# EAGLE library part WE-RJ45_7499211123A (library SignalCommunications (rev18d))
Order Code 7499211123A Design THT xBase-T 10/100 Base-T Ports 1x1 Application PoE HPLE Tab Position Down LED (Left-Right) YELLOW-GREEN EMI Fingers YES Details see: http://katalog.we-online.de/en/pbs/WE-LAN_RJ45/7499211123A? Updated by Yingchun Shan 2016-08-30 2016(C) Würth Elektronik
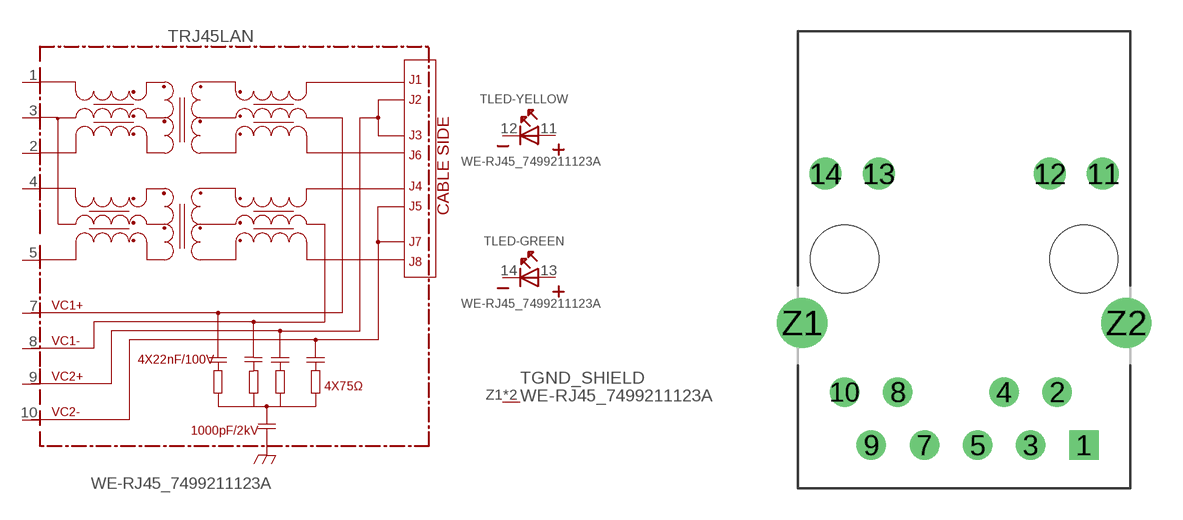
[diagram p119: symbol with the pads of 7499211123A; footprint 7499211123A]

Designator prefix T; gates RJ45LAN=7499211123A LED-YELLOW=LED-2PIN LED-GREEN=LED-2PIN GND_SHIELD=GND_PIN

## WE-RJ45_7499211123A (COMPANY-URL: http://www.we-online.de; CREATED-BY: Christin Zierenner; CREATED-DATE: AUG 2012; DATASHEET-URL: http://katalog.we-online.de/pbs/datasheet/7499211123A.pdf; MANUFACTURER: Würth Elektronik eiSos GmbH)  [7499211123A]
1  RJ45LAN:1
2  RJ45LAN:2
3  RJ45LAN:3
4  RJ45LAN:4
5  RJ45LAN:5
7  RJ45LAN:VC1+  pwr
8  RJ45LAN:VC1-  pwr
9  RJ45LAN:VC2+  pwr
10  RJ45LAN:VC2-  pwr
11  LED-YELLOW:A  pas
12  LED-YELLOW:K  pas
13  LED-GREEN:A  pas
14  LED-GREEN:K  pas
Z1  GND_SHIELD:1  pwr
Z2  GND_SHIELD:1  pwr

## Footprint 7499211123A (pad centres in mm)
MAX HEIGHT=13.95mm PORTS----1X1 LED --YES
drill 0.9 square: 1 5.715,-8.89
drill 0.9: 2 4.445,-6.35; 3 3.175,-8.89; 4 1.905,-6.35; 5 0.635,-8.89; 7 -1.905,-8.89; 8 -3.175,-6.35; 9 -4.445,-8.89; 10 -5.715,-6.35
drill 1.02: 11 6.63,4.08; 12 4.09,4.08; 13 -4.09,4.08; 14 -6.63,4.08
drill 1.6: Z1 -7.745,-3.05; Z2 7.745,-3.05
hole 3.25 at 5.715,0
hole 3.25 at -5.715,0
